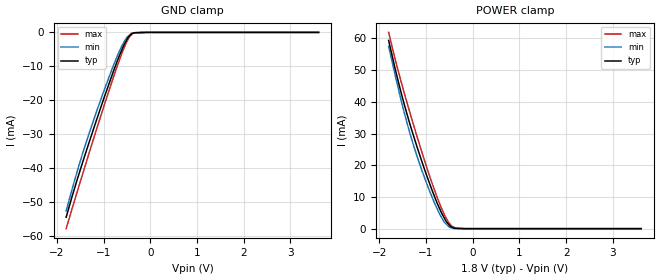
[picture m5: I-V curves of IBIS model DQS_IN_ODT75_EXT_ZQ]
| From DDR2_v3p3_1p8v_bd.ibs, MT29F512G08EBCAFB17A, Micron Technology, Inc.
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| MODEL DQS_IN_ODT75_EXT_ZQ (Data Strobe Input with 75ohm ODT, With ZQ Cal)
[Model]   DQS_IN_ODT75_EXT_ZQ
Model_type   Input
Vinl = 650.000mV
Vinh = 1.150V
|   typ   min   max
|C_comp   1.136pF   1.026pF   1.246pF
C_comp_power_clamp   0.5680pF   0.5130pF   0.6230pF
C_comp_gnd_clamp   0.5680pF   0.5130pF   0.6230pF
| Note: C_comp changes when the ODT circuit is enabled.
[Model Spec]
| Input threshold voltage corners
Vinl   0.6500V   0.6000V   0.7250V
Vinh   1.1500V   1.1000V   1.2250V
| Dynamic Overshoot Parameters from ONFI4 Specification
D_overshoot_ampl_h   1.00   NA   NA
D_overshoot_ampl_l   1.00   NA   NA
D_overshoot_area_h   0.75n   NA   NA
D_overshoot_area_l   0.75n   NA   NA
[Receiver Thresholds]
|Vth   =  0.900V
|Vth_min  =  0.8820V
|Vth_max  =  0.9180V
|Vinh_ac  =  0.250V
|Vinh_dc  =  0.125V
|Vinl_ac  = -0.250V
|Vinl_dc  = -0.125V
|Tslew_ac =  5.000ns |Not specified, so set to high value
|Threshold_sensitivity = 0.50
|Reference_supply Power_clamp_ref
Vcross_low   = 0.725V
Vcross_high  = 1.075V
Vdiff_ac   = 500mV
Vdiff_dc   = 250mV
Tdiffslew_ac = 10.000ns |Not specified, so set to high value
[Voltage Range]   1.8000V   1.7000V   1.9500V
[POWER Clamp Reference]   1.8000V   1.7000V   1.9500V
| Junction Temperature (Ambient temp is 35C typ, 70C min, 0C max)
[Temperature Range]   50.0   85.0   0.0
[Add Submodel]
| Submodel Name   Mode
75ohm_ODT_EXT_ZQ   Non-Driving
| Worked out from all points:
|   GND clamp passes 1 mA (typ) near -0.44 V on its own axis
|   POWER clamp passes 1 mA (typ) near -0.50 V on its own axis
[GND Clamp]
|   Voltage   I(typ)   I(min)   I(max)
-1.8V     -54.56mA   -52.69mA   -57.93mA
-1.548V   -42.78mA   -40.31mA   -46.36mA
-1.327V   -33.25mA   -30.57mA   -36.44mA
-1.077V   -22.86mA   -20.51mA   -25.43mA
-817.4mV  -12.62mA   -10.81mA   -14.45mA
-608.3mV  -5.168mA   -3.972mA   -6.219mA
-520.8mV  -2.645mA   -1.885mA   -3.256mA
-480.6mV  -1.611mA   -1.209mA   -2.217mA
-442.8mV  -1.066mA   -762.6uA   -1.241mA
-364.8mV  -238.2uA   -221uA     -173.5uA
-163.8mV  -972.9nA   0A         -201.1uA
3.604V    0A         0A         0A
[POWER Clamp]
|   Voltage   I(typ)   I(min)   I(max)
-1.8V     59.37mA    57.52mA    61.9mA
-1.585V   45.91mA    43.7mA     49.21mA
-1.437V   37.69mA    35mA       41.3mA
-1.276V   29.7mA     26.71mA    33.17mA
-1.077V   20.68mA    17.92mA    23.6mA
-871.2mV  12.13mA    9.982mA    14.37mA
-712mV    6.399mA    4.675mA    8.008mA
-572.4mV  2.368mA    1.496mA    3.424mA
-504.6mV  1.145mA    486.6uA    1.765mA
-442.8mV  468.7uA    231.8uA    685.7uA
-178.2mV  0A         0A         0A
3.604V    0A         0A         0A
